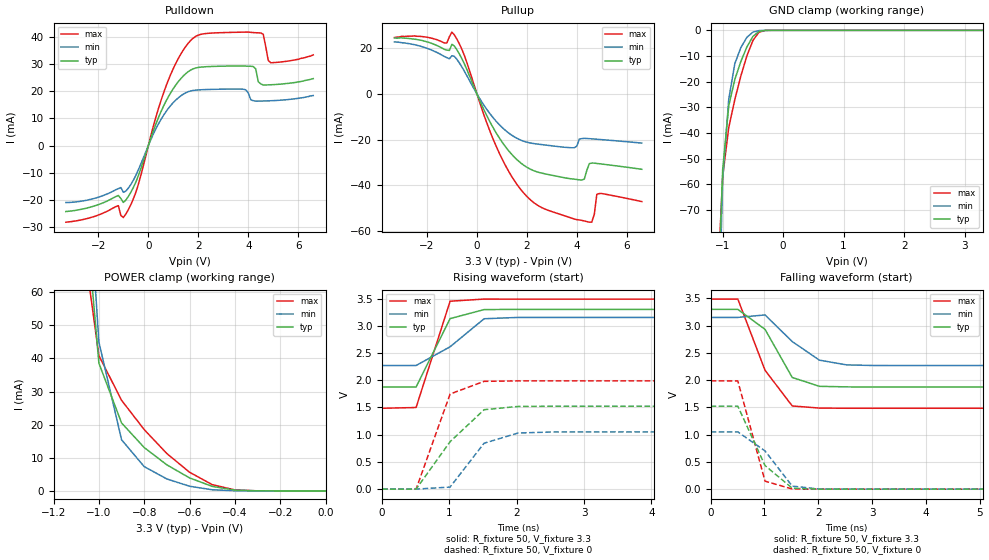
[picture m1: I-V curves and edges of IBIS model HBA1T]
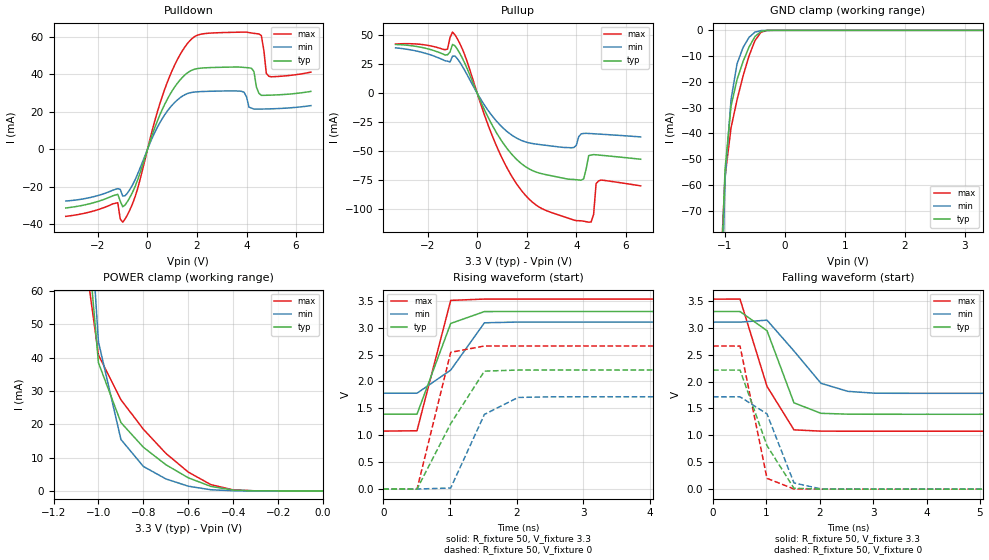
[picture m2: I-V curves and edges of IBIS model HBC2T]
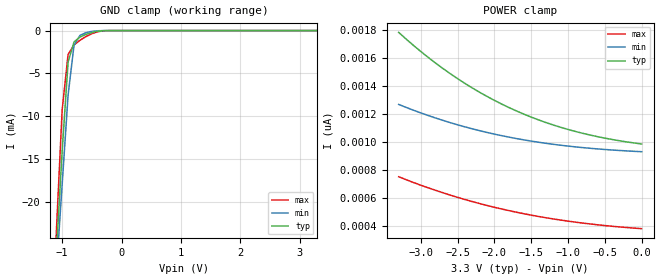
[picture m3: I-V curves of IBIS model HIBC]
[IBIS Ver]   3.2
[Comment Char]   |_char
[File name]   S1D13517.ibs
[File Rev]   1.0
[Date]   2013/01/31
[Source]
[Notes]
[Disclaimer]
This information is for modeling purposes only, and is not guaranteed.
Property of SEIKO EPSON Corp.,
unauthorized reproduction and/or distribution is strictly prohibited.
[Copyright]
Copyright 2013, SEIKO EPSON Corp.
[Component]   S1D13517
Si_location Pin
Timing_location Pin
[Manufacturer]   SEIKO EPSON Corp.
| QFP15-128
| QFP15-128
[Package]
R_pkg   155.46m   147.99m   164.96m
L_pkg   1.91n   1.54n   2.28n
C_pkg   0.77p   0.73p   0.82p
[Pin] signal_name   model_name
1   VSS   GND
2   HD3   HBA1T
3   HD4   HBA1T
4   HD5   HBA1T
5   HD6   HBA1T
6   HD7   HBA1T
7   HD8   HBA1T
8   HD9   HBA1T
9   HD10   HBA1T
10   HD11   HBA1T
11   HD12   HBA1T
12   HD13   HBA1T
13   HD14   HBA1T
14   HD15   HBA1T
15   LVDD   POWER
16   HVDD   POWER
17   VSS   GND
18   CLKI   HIBC
19   TEST0   ITST1
20   TEST1   HIBCD2
21   CNF2   HIBC
22   CNF1   HIBC
23   CNF0   HIBC
24   MVSS   GND
25   MVDD   POWER
26   PLLCHGO   LOT
27   AVDD   POWER
28   AVSS   GND
29   RESET#   HIBH
30   SCANEN   HIBCD2
31   HVDD   POWER
32   VSS   GND
33   MA3   HOB2T
34   MA4   HOB2T
35   MA2   HOB2T
36   MA5   HOB2T
37   MA1   HOB2T
38   MA6   HOB2T
39   MA0   HOB2T
40   MA7   HOB2T
41   MA10   HOB2T
42   MA8   HOB2T
43   MBA1   HOB2T
44   MA9   HOB2T
45   MBA0   HOB2T
46   MA11   HOB2T
47   HVDD   POWER
48   VSS   GND
49   MCS#   HOB2T
50   MCKE   HOB2T
51   MRAS#   HOB2T
52   LVDD   POWER
53   MCLKI   HIBC
54   VSS   GND
55   MCLKO   HOB3AT
56   MCAS#   HOB2T
57   MDQM1   HOB2T
58   MWE#   HOB2T
59   MDQM0   HOB2T
60   MD7   HBC2T
61   MD8   HBC2T
62   MD6   HBC2T
63   MD9   HBC2T
64   HVDD   POWER
65   VSS   GND
66   MD5   HBC2T
67   MD10   HBC2T
68   MD4   HBC2T
69   MD11   HBC2T
70   MD3   HBC2T
71   MD12   HBC2T
72   MD2   HBC2T
73   MD13   HBC2T
74   MD1   HBC2T
75   MD14   HBC2T
76   MD0   HBC2T
77   MD15   HBC2T
78   LVDD   POWER
79   HVDD   POWER
80   VSS   GND
81   PDE   HOB1T
82   PVS   HOB1T
83   PHS   HOB1T
84   PD_B7   HOB1T
85   PD_B6   HOB1T
86   PD_B5   HOB1T
87   PD_B4   HOB1T
88   PD_B3   HOB1T
89   PD_B2   HOB1T
90   PD_B1   HOB1T
91   PD_B0   HOB1T
92   PD_G7   HOB1T
93   PD_G6   HOB1T
94   PD_G5   HOB1T
95   PD_G4   HOB1T
96   HVDD   POWER
97   VSS   GND
98   PD_G3   HOB1T
99   PD_G2   HOB1T
100   PD_G1   HOB1T
101   PD_G0   HOB1T
102   PD_R7   HOB1T
103   PD_R6   HOB1T
104   PD_R5   HOB1T
105   PD_R4   HOB1T
106   PD_R3   HOB1T
107   PD_R2   HOB1T
108   PD_R1   HOB1T
109   PD_R0   HOB1T
110   PCLK   HOB1T
111   GPO3   HOB1T
112   LVDD   POWER
113   HVDD   POWER
114   VSS   GND
115   GPO2   HOB1T
116   GPO1   HOB1T
117   GPO0   HOB1T
118   PWM   HOB1T
119   TE   HOB1T
120   HDC#   HIBC
121   HALE   HIBC
122   HWE#   HIBH
123   HCS#   HIBC
124   HRE#   HIBC
125   HD0   HBA1T
126   HD1   HBA1T
127   HD2   HBA1T
128   HVDD   POWER
| Models and submodels in the file (10): HBA1T (I/O), HBC2T (I/O), HIBC (Input), HIBCD2 (Input), HIBH (Input), HOB1T (Output), HOB2T (Output), HOB3AT (Output), ITST1 (Input), LOT (Output)
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[Model]   HBA1T
Model_type I/O
Enable Active-Low
Polarity Non-Inverting
C_comp   5p   4p   6p
[Temperature Range] 50   100   0
[Voltage Range]   3.3   3.0   3.6
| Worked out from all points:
|   slope of the pulldown table from 0 to 0.495 V, typ, clamps not added: 40.4 ohm
|   slope of the pullup table from 0 to 0.495 V, typ, clamps not added: 42.4 ohm
|   GND clamp passes 1 mA (typ) near -0.43 V on its own axis
|   POWER clamp passes 1 mA (typ) near -0.47 V on its own axis
|   falling waveform, R_fixture 50, V_fixture 3.3: 20-80 % time 555ps typ, 665ps min, 579ps max; typ from 3.3 V to 1.88 V
|   falling waveform, R_fixture 50, V_fixture 0: 20-80 % time 519ps typ, 584ps min, 327ps max; typ from 1.52 V to 0 V
|   rising waveform, R_fixture 50, V_fixture 3.3: 20-80 % time 344ps typ, 602ps min, 311ps max; typ from 1.88 V to 3.3 V
|   rising waveform, R_fixture 50, V_fixture 0: 20-80 % time 627ps typ, 395ps min, 345ps max; typ from 0 V to 1.52 V
[Pullup]
-3.3V     24.48mA    22.74mA    24.65mA
-1.2V     19.16mA    15.83mA    22.29mA
-900mV    20.89mA    16.4mA     25.77mA
1V        -20.97mA   -14.6mA    -28.3mA
1.7V      -29.74mA   -19.97mA   -41.07mA
2.4V      -34.12mA   -21.95mA   -48.56mA
3.9V      -37.33mA   -23.58mA   -54.78mA
4.2V      -37.75mA   -19.6mA    -55.39mA
4.5V      -30.52mA   -19.62mA   -56.18mA
4.7V      -30.33mA   -19.79mA   -52.72mA
4.8V      -30.46mA   -19.87mA   -43.99mA
6.6V      -33.02mA   -21.56mA   -47.15mA
[Pulldown]
-3.3V     -24.24mA   -20.91mA   -28.16mA
-1.2V     -18.34mA   -15.83mA   -22.07mA
-1.1V     -19.46mA   -15.42mA   -25.67mA
-900mV    -20.04mA   -16.72mA   -25.18mA
-400mV    -11.05mA   -8.882mA   -14.26mA
800mV     17.95mA    13.68mA    24.09mA
1.9V      28.56mA    20.41mA    40.22mA
3.8V      29.29mA    20.75mA    41.74mA
4.2V      29.07mA    16.54mA    41.59mA
4.5V      22.72mA    16.39mA    41.43mA
4.9V      22.39mA    16.51mA    30.48mA
6.6V      24.66mA    18.42mA    33.38mA
[GND Clamp]
-3.3V     -3.904A    -3.557A    -4.353A
-1.1V     -118.9mA   -145mA     -106mA
-1V       -54.09mA   -58.05mA   -56.96mA
-900mV    -29.42mA   -26.86mA   -37.89mA
-800mV    -19.16mA   -13.01mA   -27.02mA
-700mV    -12.15mA   -6.718mA   -17.78mA
-600mV    -6.477mA   -2.726mA   -9.93mA
-500mV    -2.365mA   -667.1uA   -3.94mA
-400mV    -431.6uA   -96.18uA   -746.4uA
-300mV    -40.31uA   -9.839uA   -57.18uA
3.3V      5.041nA    4.638uA    977pA
[POWER Clamp]
-3.3V     3.948A     3.603A     4.377A
-1.1V     117.5mA    151.4mA    91.09mA
-1V       38.6mA     44.98mA    40.87mA
-900mV    20.53mA    15.46mA    27.37mA
-800mV    13.1mA     7.338mA    18.51mA
-700mV    7.867mA    3.611mA    11.28mA
-600mV    3.929mA    1.414mA    5.638mA
-500mV    1.368mA    349.4uA    1.9mA
-400mV    257.4uA    50.44uA    302.5uA
-300mV    26.21uA    4.639uA    23.79uA
0V        5.041nA    5.145nA    1.201nA
[Falling Waveform]
R_fixture=50
V_fixture=3.3
0s        3.3V       3.152V     3.489V
505.1ps   3.3V       3.152V     3.489V
1.01ns    2.933V     3.198V     2.182V
1.515ns   2.05V      2.709V     1.527V
2.02ns    1.887V     2.368V     1.488V
2.525ns   1.877V     2.281V     1.485V
3.03ns    1.875V     2.269V     1.485V
50ns      1.875V     2.269V     1.485V
[Falling Waveform]
R_fixture=50
V_fixture=0
0s        1.522V     1.05V      1.988V
505.1ps   1.522V     1.051V     1.986V
1.01ns    432.4mV    701.5mV    145.7mV
1.515ns   17.25mV    54.75mV    2.352mV
2.02ns    -862.4uV   2.265mV    70.54uV
2.525ns   124.8uV    394.4uV    -1.129uV
50ns      11.44uV    11.07uV    -10.52uV
[Rising Waveform]
R_fixture=50
V_fixture=3.3
0s        1.875V     2.269V     1.485V
505.1ps   1.875V     2.27V      1.498V
1.01ns    3.131V     2.614V     3.45V
1.515ns   3.297V     3.128V     3.49V
2.02ns    3.3V       3.153V     3.488V
50ns      3.3V       3.152V     3.489V
[Rising Waveform]
R_fixture=50
V_fixture=0
0s        0V         0V         0V
505.1ps   10.33uV    -1.968uV   -964.5uV
1.01ns    870.3mV    37.34mV    1.746V
1.515ns   1.458V     843.2mV    1.979V
2.02ns    1.518V     1.031V     1.988V
2.525ns   1.522V     1.049V     1.988V
50ns      1.522V     1.05V      1.988V
[Ramp]
R_load=50
dV/dt_r   9.131E-1/3.230E-10   6.301E-1/3.883E-10   1.193E+0/2.630E-10
dV/dt_f   8.550E-1/4.054E-10   6.142E-1/4.911E-10   1.155E+0/3.391E-10
|[End   HBA1T
[Model]   HBC2T
Model_type I/O
Enable Active-Low
Polarity Non-Inverting
C_comp   5p   4p   6p
[Temperature Range] 50   100   0
[Voltage Range]   3.3   3.0   3.6
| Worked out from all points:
|   slope of the pulldown table from 0 to 0.495 V, typ, clamps not added: 27.1 ohm
|   slope of the pullup table from 0 to 0.495 V, typ, clamps not added: 21.5 ohm
|   GND clamp passes 1 mA (typ) near -0.43 V on its own axis
|   POWER clamp passes 1 mA (typ) near -0.47 V on its own axis
|   falling waveform, R_fixture 50, V_fixture 3.3: 20-80 % time 431ps typ, 679ps min, 566ps max; typ from 3.3 V to 1.39 V
|   falling waveform, R_fixture 50, V_fixture 0: 20-80 % time 579ps typ, 405ps min, 328ps max; typ from 2.21 V to 0 V
|   rising waveform, R_fixture 50, V_fixture 3.3: 20-80 % time 343ps typ, 555ps min, 307ps max; typ from 1.39 V to 3.3 V
|   rising waveform, R_fixture 50, V_fixture 0: 20-80 % time 608ps typ, 380ps min, 317ps max; typ from 0 V to 2.21 V
[Pullup]
-3.3V     42.15mA    39.25mA    42.56mA
-1.3V     33.08mA    28.08mA    37.61mA
-900mV    41.01mA    32.19mA    50.49mA
1V        -41.53mA   -29.01mA   -55.83mA
2.5V      -68.74mA   -44.13mA   -98.09mA
3.9V      -74.3mA    -46.75mA   -109.3mA
4.2V      -74.89mA   -34.96mA   -110mA
4.6V      -53.23mA   -34.74mA   -111mA
4.7V      -52.84mA   -34.87mA   -104.3mA
4.8V      -53.04mA   -35mA      -77.92mA
4.9V      -53.23mA   -35.13mA   -75.58mA
6.6V      -56.86mA   -37.58mA   -79.82mA
[Pulldown]
-3.3V     -31.32mA   -27.59mA   -35.8mA
-1.2V     -24.05mA   -20.99mA   -28.51mA
-1.1V     -27.67mA   -21.42mA   -37.18mA
-900mV    -29.63mA   -24.72mA   -37.13mA
-400mV    -16.4mA    -13.21mA   -21.1mA
800mV     26.75mA    20.42mA    35.8mA
1.9V      42.8mA     30.61mA    60.2mA
3.8V      43.88mA    31mA       62.61mA
4.2V      43.29mA    22.07mA    62.14mA
4.5V      29.94mA    21.51mA    61.64mA
4.9V      28.92mA    21.61mA    39.05mA
6.6V      30.96mA    23.36mA    41.27mA
[GND Clamp]
-3.3V     -3.834A    -3.499A    -4.267A
-1.1V     -117.7mA   -143.2mA   -105.3mA
-1V       -53.96mA   -57.85mA   -56.85mA
-900mV    -29.39mA   -26.83mA   -37.84mA
-800mV    -19.14mA   -13mA      -26.98mA
-700mV    -12.14mA   -6.714mA   -17.76mA
-600mV    -6.473mA   -2.725mA   -9.921mA
-500mV    -2.364mA   -667uA     -3.937mA
-400mV    -431.6uA   -96.18uA   -746.3uA
-300mV    -40.31uA   -9.839uA   -57.18uA
3.3V      5.147nA    4.638uA    954.9pA
[POWER Clamp]
-3.3V     3.869A     3.537A     4.281A
-1.1V     115.6mA    148.9mA    90mA
-1V       38.44mA    44.67mA    40.76mA
-900mV    20.5mA     15.43mA    27.33mA
-800mV    13.09mA    7.333mA    18.49mA
-700mV    7.862mA    3.61mA     11.27mA
-600mV    3.928mA    1.413mA    5.634mA
-500mV    1.368mA    349.4uA    1.9mA
-400mV    257.4uA    50.44uA    302.4uA
-300mV    26.21uA    4.638uA    23.79uA
0V        5.147nA    5.009nA    1.16nA
[Falling Waveform]
R_fixture=50
V_fixture=3.3
0s        3.3V       3.103V     3.531V
505.1ps   3.3V       3.103V     3.532V
1.01ns    2.945V     3.14V      1.91V
1.515ns   1.604V     2.568V     1.102V
2.02ns    1.409V     1.967V     1.078V
2.525ns   1.393V     1.817V     1.077V
3.03ns    1.392V     1.783V     1.077V
50ns      1.391V     1.781V     1.077V
[Falling Waveform]
R_fixture=50
V_fixture=0
0s        2.212V     1.715V     2.659V
505.1ps   2.212V     1.716V     2.659V
1.01ns    808.5mV    1.398V     201.2mV
1.515ns   16.42mV    115.1mV    2.424mV
2.02ns    1.162mV    4.637mV    54.99uV
2.525ns   -208.8uV   474.8uV    -55.04uV
50ns      -7.678uV   -1.051uV   -12.68uV
[Rising Waveform]
R_fixture=50
V_fixture=3.3
0s        1.391V     1.781V     1.077V
505.1ps   1.391V     1.781V     1.084V
1.01ns    3.078V     2.211V     3.507V
1.515ns   3.299V     3.09V      3.531V
2.02ns    3.3V       3.104V     3.531V
50ns      3.3V       3.103V     3.531V
[Rising Waveform]
R_fixture=50
V_fixture=0
0s        0V         0V         0V
505.1ps   12.4uV     -4.607uV   -2.062mV
1.01ns    1.216V     19.63mV    2.541V
1.515ns   2.192V     1.387V     2.659V
2.02ns    2.212V     1.703V     2.659V
2.525ns   2.212V     1.715V     2.659V
50ns      2.212V     1.715V     2.659V
[Ramp]
R_load=50
dV/dt_r   1.327E+0/2.569E-10   1.029E+0/3.456E-10   1.595E+0/1.857E-10
dV/dt_f   1.145E+0/3.818E-10   8.802E-1/5.159E-10   1.437E+0/2.869E-10
|[End   HBC2T
[Model]   HIBC
Model_type Input
C_comp   5p   4p   6p
[Temperature Range] 50   100   0
[Voltage Range]   3.3   3.0   3.6
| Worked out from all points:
|   GND clamp passes 1 mA (typ) near -0.74 V on its own axis
[GND Clamp]
-3.3V     -310.4mA   -271.5mA   -364.3mA
-1.1V     -26.25mA   -28.4mA    -23.85mA
-1V       -14.07mA   -17.95mA   -9.285mA
-900mV    -3.667mA   -7.529mA   -2.767mA
-800mV    -1.326mA   -1.694mA   -1.687mA
-700mV    -753.9uA   -566.6uA   -1.131mA
-600mV    -445.2uA   -244.2uA   -699.4uA
-500mV    -223.9uA   -92.7uA    -365.2uA
-300mV    -11.88uA   -2.451uA   -21.75uA
3.3V      985.3pA    938.7pA    367.6pA
[POWER Clamp]
-3.3V     1.786nA    1.269nA    750.1pA
-3V       1.649nA    1.208nA    689.7pA
-2.8V     1.566nA    1.172nA    652.8pA
-2.6V     1.49nA     1.139nA    618.5pA
-2.4V     1.42nA     1.108nA    586.9pA
-2.2V     1.356nA    1.081nA    557.8pA
-2V       1.298nA    1.056nA    531.1pA
-1.8V     1.246nA    1.034nA    506.9pA
-1.4V     1.158nA    997.9pA    465.1pA
-1V       1.09nA     970.3pA    431.7pA
-500mV    1.027nA    946pA      400.1pA
0V        985.3pA    929.8pA    377.7pA
